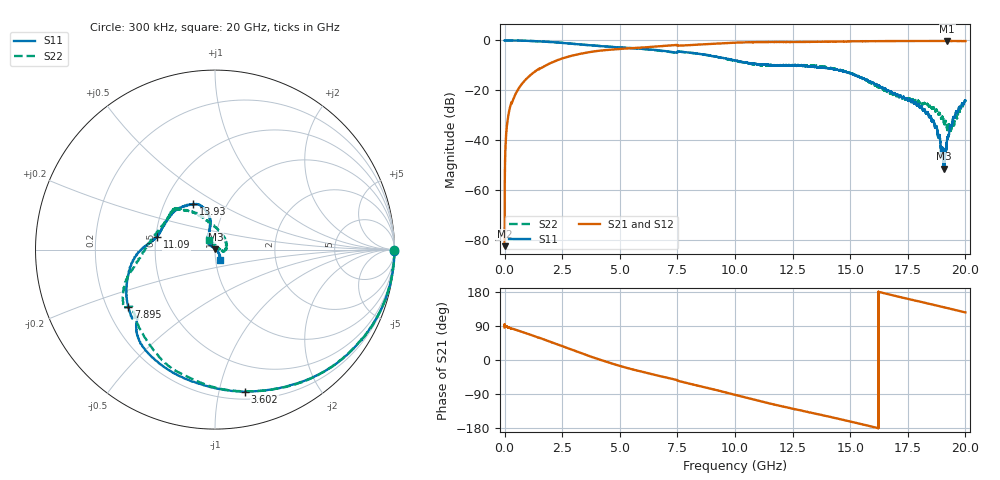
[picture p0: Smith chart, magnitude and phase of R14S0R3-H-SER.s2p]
!{R14S0R3}
!Johanson Technology Inc.
!www.johansontechnology.com
!Test Board Conditions:
!Substrate Type  RO4350B
!Substrate Thickness  20 mil
!Substrate Dk  3.66
!TL Type: GCPW
!TL Trace Width  36 mil
!TL Gap  12 mil
!Electrode orientation  Horizontal
!DUT TOPOLOGY	SERIES
!Mounting Pad LxW  26x36 mil
! Created Wed Nov 25 17:33:21 2020
! 2 Port Network Data from SP1.SP block
! freq  magS11  angS11  magS21  angS21  magS12  angS12  magS22  angS22
# khz S ma R 50
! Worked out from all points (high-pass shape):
!   20001 points, 300 kHz to 20 GHz, reference 50 ohm
!   highest |S21| = -0.19 dB at 19.2 GHz (marker M1); lowest = -82.4 dB at 300 kHz (marker M2)
!   |S21| within 3 dB of the highest: 5.320251 GHz to 5.322054 GHz (1.804 MHz wide, 0.0339 % of centre); 5.326 GHz to end of sweep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
!   lowest |S11| = -51.3 dB at 19.07 GHz (marker M3), VSWR 1.01, Z = 50.3 + j0.0839 ohm
!   |S11| at or under -10 dB: 12.35 GHz to 12.49 GHz (136.3 MHz wide, 1.1 % of centre); 12.5 GHz to 12.6 GHz (96.31 MHz wide, 0.768 % of centre); 12.62 GHz to end of sweep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
!   |S22| runs from -36.3 to 0.0 dB; largest |S21 - S12| = 0.014
!   S11 on the Smith chart (normalised r, x): 300 kHz: open; 3.602 GHz: 0.26, -1.20; 7.895 GHz: 0.29, -0.28; 11.09 GHz: 0.51, +0.08; 13.93 GHz: 0.70, +0.38; 20 GHz: 1.05, -0.12
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300  0.9966 -0.4  7.602e-05 85.9  0.0001273 111.6  0.9983 -0.2
102300  0.9997 -2.3  0.02001 87.5  0.02012 87.4  0.9997 -2.2
140300  0.9992 -3.0  0.02742 86.6  0.02756 86.7  0.9992 -3.0
268300  0.9973 -6.0  0.05238 83.4  0.05265 83.4  0.9984 -6.0
526300  0.9953 -10.7  0.09407 78.9  0.09427 79.1  0.9943 -10.6
1399300  0.9627 -29.5  0.2538 60.5  0.2545 60.4  0.9647 -29.4
3334300  0.8271 -72.1  0.5457 17.8  0.5466 17.8  0.8273 -72.0
3602300  0.8081 -78.1  0.5753 11.9  0.576 12.0  0.8079 -77.7
5224300  0.7149 -112.6  0.6867 -19.5  0.6871 -19.3  0.714 -106.0
6667300  0.6357 -133.3  0.761 -41.4  0.763 -41.2  0.6279 -128.3
7895300  0.5791 -146.6  0.8004 -60.5  0.8045 -60.4  0.5782 -152.9
1.00003e7  0.3995 178.3  0.9009 -91.9  0.9043 -91.9  0.3909 179.5
1.10853e7  0.3295 167.5  0.9277 -108.3  0.9274 -108.7  0.3234 155.8
1.33343e7  0.299 127.4  0.938 -139.6  0.9334 -139.6  0.3115 133.7
1.39283e7  0.2811 115.7  0.9458 -147.4  0.9383 -147.5  0.2954 130.2
1.66673e7  0.09975 110.3  0.9722 173.3  0.9732 173.6  0.09418 62.3
1.84133e7  0.03006 138.0  0.9709 148.6  0.9722 148.5  0.04762 -11.1
1.86913e7  0.01826 133.5  0.9735 144.6  0.9746 144.8  0.03805 -11.8
1.90653e7  0.002722 17.9  0.9736 139.2  0.9763 139.2  0.02275 8.5
1.92043e7  0.01012 -32.8  0.9781 137.2  0.9746 137.2  0.0172 28.0
1.95313e7  0.02859 -39.8  0.9735 132.4  0.974 132.3  0.02309 80.5
2e7  0.06234 -62.9  0.9722 125.5  0.9669 125.4  0.062 123.7
